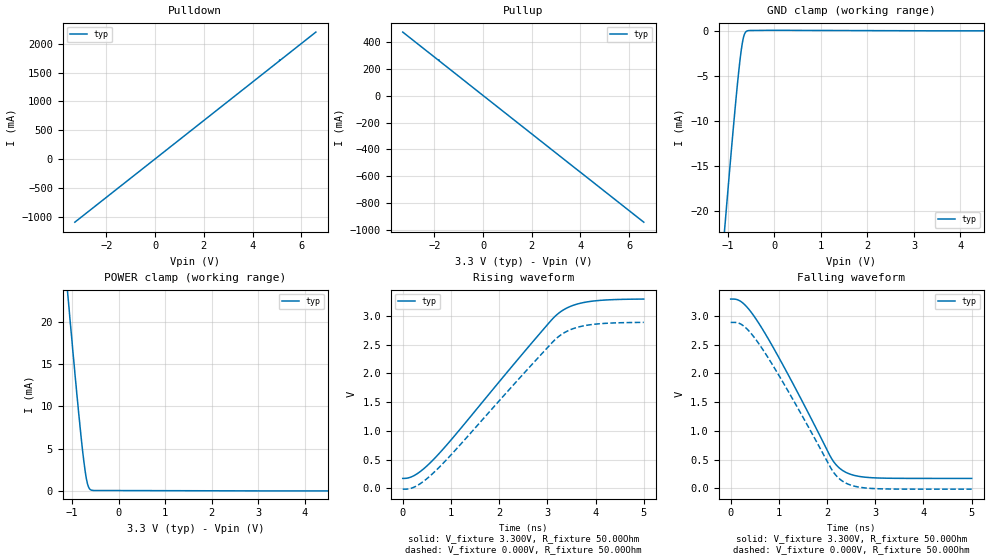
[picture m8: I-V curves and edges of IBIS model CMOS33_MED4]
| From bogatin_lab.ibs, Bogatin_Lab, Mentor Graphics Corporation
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[Model]   CMOS33_MED4
Model_type   I/O
Vinl = 800.000mV
Vinh = 2.000V
Vmeas = 1.500V
Vref = 0.000V
Cref = 50.000pF
Rref = 1.000kOhm
|   typ   min   max
C_comp   4.000pF   NA   NA
[Voltage Range]   3.300V   NA   NA
[Temperature Range]   50.0   NA   NA
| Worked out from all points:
|   slope of the pulldown table from 0 to 0.495 V, typ, clamps not added: 3 ohm
|   slope of the pullup table from 0 to 0.495 V, typ, clamps not added: 7 ohm
|   GND clamp passes 1 mA (typ) near -0.68 V on its own axis
|   POWER clamp passes 1 mA (typ) near -0.68 V on its own axis
|   falling waveform, V_fixture 3.300V, R_fixture 50.00Ohm: 20-80 % time 1.19ns typ, NA min, NA max; typ from 3.29 V to 0.175 V
|   rising waveform, V_fixture 3.300V, R_fixture 50.00Ohm: 20-80 % time 1.86ns typ, NA min, NA max; typ from 0.175 V to 3.29 V
|   rising waveform, V_fixture 0.000V, R_fixture 50.00Ohm: 20-80 % time 1.86ns typ, NA min, NA max; typ from -0.012 V to 2.88 V
|   falling waveform, V_fixture 0.000V, R_fixture 50.00Ohm: 20-80 % time 1.19ns typ, NA min, NA max; typ from 2.88 V to -0.012 V
[Pulldown]
|   Voltage   I(typ)   I(min)   I(max)
-3.3V     -1.095A    NA         NA
5.1V      1.705A     NA         NA
5.11V     1.72A      NA         NA
5.12V     1.711A     NA         NA
6.6V      2.205A     NA         NA
[GND Clamp]
|   Voltage   I(typ)   I(min)   I(max)
-3.3V     -166.6mA   NA         NA
-1.09V    -23.21mA   NA         NA
-1.05V    -20.74mA   NA         NA
-920mV    -12.89mA   NA         NA
-850mV    -8.86mA    NA         NA
-790mV    -5.64mA    NA         NA
-740mV    -3.243mA   NA         NA
-700mV    -1.684mA   NA         NA
-670mV    -834.4uA   NA         NA
-630mV    -223.1uA   NA         NA
-590mV    -22.68uA   NA         NA
6.6V      0A         NA         NA
[Pullup]
|   Voltage   I(typ)   I(min)   I(max)
-3.3V     473.4mA    NA         NA
-1.82V    261.8mA    NA         NA
-1.81V    267mA      NA         NA
-1.8V     259.1mA    NA         NA
6.6V      -940.8mA   NA         NA
[POWER Clamp]
|   Voltage   I(typ)   I(min)   I(max)
-3.3V     166.5mA    NA         NA
-1.09V    23.06mA    NA         NA
-1.08V    22.46mA    NA         NA
-990mV    16.9mA     NA         NA
-860mV    9.29mA     NA         NA
-810mV    6.553mA    NA         NA
-750mV    3.621mA    NA         NA
-710mV    2.009mA    NA         NA
-670mV    866.8uA    NA         NA
-630mV    294.3uA    NA         NA
-590mV    105.4uA    NA         NA
6.6V      0A         NA         NA
[Ramp]
R_load = 50.00Ohm
|   typ   min   max
dV/dt_r   1.739V/1.863ns   NA   NA
dV/dt_f   1.870V/1.190ns   NA   NA
[Falling Waveform]
V_fixture = 3.300V
R_fixture = 50.00Ohm
|   Time   V(typ)   V(min)   V(max)
0s        3.291V     NA         NA
136.9ps   3.28V      NA         NA
254.2ps   3.221V     NA         NA
571.9ps   2.885V     NA         NA
1.178ns   2V         NA         NA
2.077ns   543mV      NA         NA
2.292ns   330.4mV    NA         NA
2.532ns   234.4mV    NA         NA
2.889ns   188.9mV    NA         NA
5ns       174.6mV    NA         NA
[Rising Waveform]
V_fixture = 3.300V
R_fixture = 50.00Ohm
|   Time   V(typ)   V(min)   V(max)
0s        174.6mV    NA         NA
141.7ps   189.8mV    NA         NA
293.3ps   252.7mV    NA         NA
684.3ps   543.8mV    NA         NA
2.825ns   2.674V     NA         NA
3.109ns   2.947V     NA         NA
3.255ns   3.058V     NA         NA
3.509ns   3.174V     NA         NA
3.837ns   3.243V     NA         NA
5ns       3.291V     NA         NA
[Rising Waveform]
V_fixture = 0.000V
R_fixture = 50.00Ohm
|   Time   V(typ)   V(min)   V(max)
0s        -12.25mV   NA         NA
151.5ps   -1.805mV   NA         NA
303ps     52.11mV    NA         NA
698.9ps   320.8mV    NA         NA
2.859ns   2.317V     NA         NA
3.138ns   2.568V     NA         NA
3.285ns   2.67V      NA         NA
3.534ns   2.776V     NA         NA
3.856ns   2.84V      NA         NA
5ns       2.885V     NA         NA
[Falling Waveform]
V_fixture = 0.000V
R_fixture = 50.00Ohm
|   Time   V(typ)   V(min)   V(max)
0s        2.885V     NA         NA
146.6ps   2.878V     NA         NA
259ps     2.829V     NA         NA
576.7ps   2.524V     NA         NA
1.178ns   1.711V     NA         NA
2.092ns   334.9mV    NA         NA
2.312ns   131.8mV    NA         NA
2.551ns   43.03mV    NA         NA
2.903ns   1.277mV    NA         NA
5ns       -12.25mV   NA         NA
